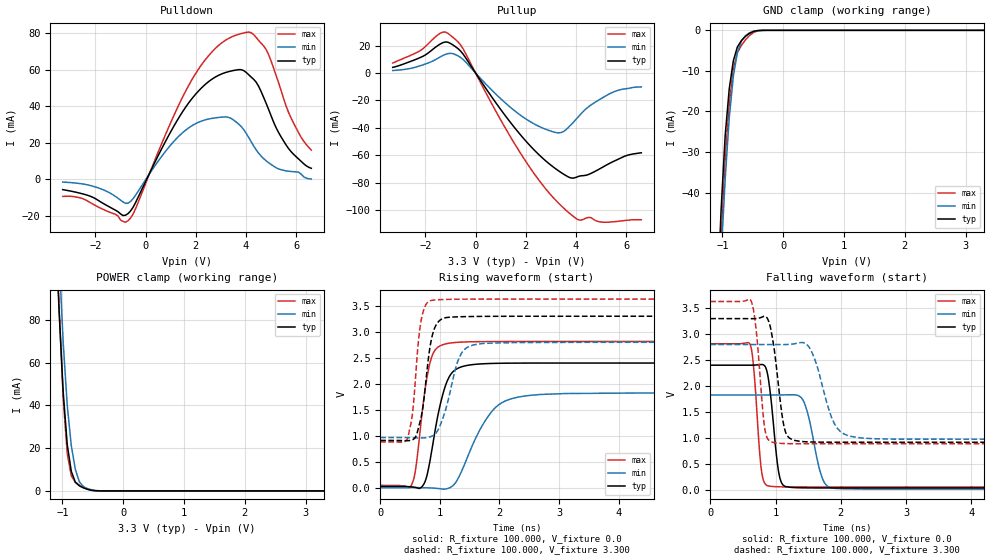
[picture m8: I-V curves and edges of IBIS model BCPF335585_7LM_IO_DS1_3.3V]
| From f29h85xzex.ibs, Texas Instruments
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|   Model BCPF335585_7LM_IO_DS1_3.3V
[Model]   BCPF335585_7LM_IO_DS1_3.3V
Model_type   I/O
Polarity   Non-Inverting
Enable   Active-Low
Vinl =   0.800V
Vinh =   2.000V
Vmeas =  1.650V
Cref =   15.000pF
Vref =   0.0V
|   typ   min   max
C_comp   0.820pF   0.815pF   0.864pF
[Model Spec]
Vinh   2.000V   2.000V   2.000V
Vinl   0.800V   0.800V   0.800V
[Temperature Range]   25   155   -40
[Voltage Range]   3.300V   2.800V   3.630V
[Pullup Reference]   3.300V   2.800V   3.630V
[Pulldown Reference]   0.0V   0.0V   0.0V
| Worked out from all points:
|   slope of the pulldown table from 0 to 0.495 V, typ, clamps not added: 35.3 ohm
|   slope of the pullup table from 0 to 0.495 V, typ, clamps not added: 36.6 ohm
|   GND clamp passes 1 mA (typ) near -0.58 V on its own axis
|   POWER clamp passes 1 mA (typ) near -0.61 V on its own axis
|   rising waveform, R_fixture 100.000, V_fixture 0.0: 20-80 % time 251ps typ, 482ps min, 185ps max; typ from 0.033 V to 2.4 V
|   rising waveform, R_fixture 100.000, V_fixture 3.300: 20-80 % time 161ps typ, 253ps min, 126ps max; typ from 0.914 V to 3.3 V
|   falling waveform, R_fixture 100.000, V_fixture 0.0: 20-80 % time 115ps typ, 184ps min, 92.9ps max; typ from 2.4 V to 0.033 V
|   falling waveform, R_fixture 100.000, V_fixture 3.300: 20-80 % time 140ps typ, 255ps min, 108ps max; typ from 3.3 V to 0.914 V
[Pulldown]
|Voltage   I(typ)   I(min)   I(max)
-3.3V     -5.694mA   -1.56mA    -9.437mA
-2V       -10.64mA   -4.236mA   -14.4mA
-700mV    -18.89mA   -13.14mA   -22.82mA
-400mV    -12.84mA   -8.81mA    -16.23mA
1V        26.01mA    18.77mA    31.05mA
1.9V      45.13mA    29.79mA    55.87mA
3.2V      58.6mA     34.18mA    76.39mA
4V        58.68mA    25.32mA    80.53mA
4.4V      53.3mA     16.17mA    77.85mA
4.8V      41.66mA    10.13mA    71.21mA
5.7V      16.72mA    4.396mA    36.42mA
6.6V      5.993mA    80uA       15.99mA
[Pullup]
|Voltage   I(typ)   I(min)   I(max)
-3.3V     4.176mA    1.868mA    7.345mA
-2.2V     11.37mA    5.369mA    16.39mA
-1.4V     21.3mA     11.87mA    29.15mA
-1.1V     22.51mA    14.23mA    28.97mA
-500mV    13.94mA    9.965mA    17.79mA
900mV     -24.04mA   -16.97mA   -30.91mA
2V        -49.57mA   -33.43mA   -64.46mA
3.1V      -68.61mA   -42.93mA   -91.01mA
3.6V      -74.81mA   -41.33mA   -100.1mA
4.1V      -75.37mA   -31.71mA   -107.1mA
5.2V      -67.21mA   -16.48mA   -108.8mA
6.6V      -58.16mA   -10.1mA    -107mA
[GND_clamp]
|Voltage   I(typ)   I(min)   I(max)
-3.3V     -1.157A    -988.6mA   -1.458A
-1.089V   -68.54mA   -77.63mA   -80.48mA
-1.022V   -44.33mA   -55.86mA   -51.42mA
-955mV    -25.99mA   -36.73mA   -31.56mA
-888mV    -14.45mA   -21.59mA   -18.26mA
-821mV    -7.535mA   -11.36mA   -9.383mA
-754mV    -4.097mA   -5.49mA    -5.515mA
-687mV    -2.502mA   -2.628mA   -3.687mA
-553mV    -723.8uA   -607.5uA   -1.252mA
-419mV    -57.46uA   -69.83uA   -143.6uA
-285mV    -1.004uA   -3.695uA   -2.412uA
3.3V      0A         0A         0A
[POWER_clamp]
|Voltage   I(typ)   I(min)   I(max)
-3.3V     2.015A     2.235A     2.186A
-1.122V   129.6mA    158mA      137.2mA
-1.055V   84.19mA    110mA      86.31mA
-988mV    46.52mA    69.72mA    43.72mA
-921mV    21.67mA    40.06mA    17.56mA
-854mV    9.159mA    21.2mA     7.031mA
-787mV    4.017mA    9.985mA    4.074mA
-720mV    2.344mA    4.225mA    2.739mA
-653mV    1.421mA    1.97mA     1.651mA
-519mV    296.8uA    519.1uA    270.8uA
-318mV    2.374uA    16.61uA    1.127uA
3.3V      0A         0A         0A
[Ramp]
| variable   typ   min   max
dV/dt_r   1.421/0.251n   1.090/0.483n   1.657/0.186n
dV/dt_f   1.430/0.140n   1.097/0.255n   1.646/0.109n
R_load = 100.000
[Rising Waveform]
R_fixture= 100.000
V_fixture= 0.0
V_fixture_min= 0.0
V_fixture_max= 0.0
|time   V(typ)   V(min)   V(max)
0s        32.96mV    9.842mV    52.53mV
522ps     25.11mV    10.67mV    54.73mV
591ps     13.2mV     10.6mV     344mV
712ps     44.93mV    8.871mV    1.546V
832ps     508.7mV    4.564mV    2.393V
1.085ns   1.936V     -18.42mV   2.765V
1.315ns   2.307V     204.7mV    2.8V
1.865ns   2.393V     1.461V     2.813V
2.295ns   2.399V     1.743V     2.813V
10ns      2.401V     1.826V     2.814V
[Rising Waveform]
R_fixture= 100.000
V_fixture= 3.300
V_fixture_min= 2.800
V_fixture_max= 3.630
|time   V(typ)   V(min)   V(max)
0s        914.4mV    970.7mV    885.5mV
464ps     911.4mV    969.2mV    979.4mV
542ps     928.8mV    967.3mV    1.447V
638ps     1.144V     964.4mV    2.792V
685ps     1.355V     963.8mV    3.211V
848ps     2.796V     988.8mV    3.6V
1.018ns   3.237V     1.242V     3.617V
1.328ns   3.288V     2.513V     3.625V
1.566ns   3.294V     2.749V     3.627V
10ns      3.298V     2.799V     3.628V
[Falling Waveform]
R_fixture= 100.000
V_fixture= 0.0
V_fixture_min= 0.0
V_fixture_max= 0.0
|time   V(typ)   V(min)   V(max)
0s        2.401V     1.826V     2.813V
613ps     2.401V     1.826V     2.795V
781ps     2.413V     1.826V     401.2mV
897ps     2.084V     1.826V     71.31mV
1.044ns   370.8mV    1.826V     55.97mV
1.147ns   61.66mV    1.828V     53.66mV
1.435ns   35.45mV    1.694V     52.57mV
1.688ns   33.65mV    332.6mV    52.49mV
1.87ns    33.35mV    30.44mV    52.48mV
10ns      32.91mV    9.856mV    52.47mV
[Falling Waveform]
R_fixture= 100.000
V_fixture= 3.300
V_fixture_min= 2.800
V_fixture_max= 3.630
|time   V(typ)   V(min)   V(max)
0s        3.298V     2.799V     3.628V
630ps     3.297V     2.799V     3.626V
837ps     3.344V     2.799V     1.166V
971ps     2.787V     2.799V     909.8mV
1.129ns   1.228V     2.798V     889.9mV
1.304ns   946.9mV    2.816V     886.3mV
1.541ns   920mV      2.693V     885.6mV
1.878ns   915.2mV    1.338V     885.5mV
2.146ns   914.6mV    1.03V      885.5mV
10ns      914.3mV    970.7mV    885.5mV
